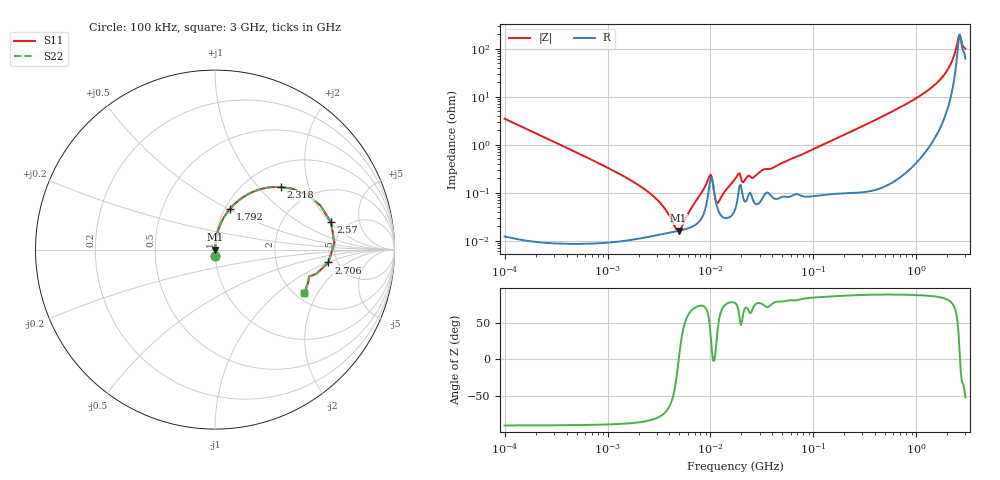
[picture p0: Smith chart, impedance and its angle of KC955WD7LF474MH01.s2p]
!Murata Part Number: KC955WD7LF474MH01
!These Parameters are Measured in Series Mode Connection
!Data Generated on Mar 13, 2026
!  o--ll--o
!Port1  Port2
!  o------o
!Operation Temp=25[degC], DC Bias Voltage=0[V]
!Freq. Start=100[kHz] Stop=3[GHz] 401[Steps]
# Hz S RI R 50
!Freq.(Hz) S11(Real) S11(Imag) S21(Real) S21(Imag) S12(Real) S12(Imag) S22(Real) S22(Imag)
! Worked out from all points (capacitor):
!   401 points, 100 kHz to 3 GHz, reference 50 ohm
!   read as one part in series: C = 458 nF near 105.3 kHz
!   lowest |Z| = 16.1 mohm at 4.899 MHz (marker M1)
!   series resonance near 4.919 MHz, so ESL is about 2.3 nH
!   S11 on the Smith chart (normalised r, x): 100 kHz: 1.00, -0.07; 1.792 GHz: 1.06, +0.51; 2.318 GHz: 1.42, +1.33; 2.57 GHz: 3.75, +2.06; 2.706 GHz: 4.23, -1.02; 3 GHz: 2.24, -1.56
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100000  0.00133 -0.0347  0.9987 0.0347  0.9987 0.0347  0.00133 -0.0347
562235  0.000123 -0.0061  0.9999 0.0061  0.9999 0.0061  0.000123 -0.0061
1747435  0.000108 -0.00173  0.9999 0.00173  0.9999 0.00173  0.000108 -0.00173
3161081  0.000133 -0.000641  0.9999 0.000641  0.9999 0.000641  0.000133 -0.000641
4899066  0.000161 -5.9e-06  0.9998 5.9e-06  0.9998 5.9e-06  0.000161 -5.9e-06
9824692  0.00152 0.00165  0.9985 -0.00165  0.9985 -0.00165  0.00152 0.00165
1.034438e7  0.002 0.000365  0.998 -0.000365  0.998 -0.000365  0.002 0.000365
1.117591e7  0.000718 0.000107  0.9993 -0.000107  0.9993 -0.000107  0.000718 0.000107
1.176708e7  0.000459 0.000401  0.9995 -0.000401  0.9995 -0.000401  0.000459 0.000401
1.77727e7  0.000533 0.00201  0.9995 -0.00201  0.9995 -0.00201  0.000533 0.00201
1.871281e7  0.000992 0.00227  0.999 -0.00227  0.999 -0.00227  0.000992 0.00227
2.128644e7  0.000678 0.00161  0.9993 -0.00161  0.9993 -0.00161  0.000678 0.00161
2.616047e7  0.000674 0.00196  0.9993 -0.00196  0.9993 -0.00196  0.000674 0.00196
9.738194e7  0.000902 0.00786  0.9991 -0.00786  0.9991 -0.00786  0.000902 0.00786
5.475153e8  0.00359 0.0457  0.9964 -0.0457  0.9964 -0.0457  0.00359 0.0457
1.156079e9  0.0185 0.1111  0.9815 -0.1111  0.9815 -0.1111  0.0185 0.1111
1.7917e9  0.084 0.2275  0.916 -0.2275  0.916 -0.2275  0.084 0.2275
2.091327e9  0.1882 0.3108  0.8118 -0.3108  0.8118 -0.3108  0.1882 0.3108
2.318426e9  0.3661 0.3494  0.6339 -0.3494  0.6339 -0.3494  0.3661 0.3494
2.570185e9  0.6455 0.1539  0.3545 -0.1539  0.3545 -0.1539  0.6455 0.1539
2.706139e9  0.6317 -0.0716  0.3683 0.0716  0.3683 0.0716  0.6317 -0.0716
3e9  0.4984 -0.2418  0.5016 0.2418  0.5016 0.2418  0.4984 -0.2418
